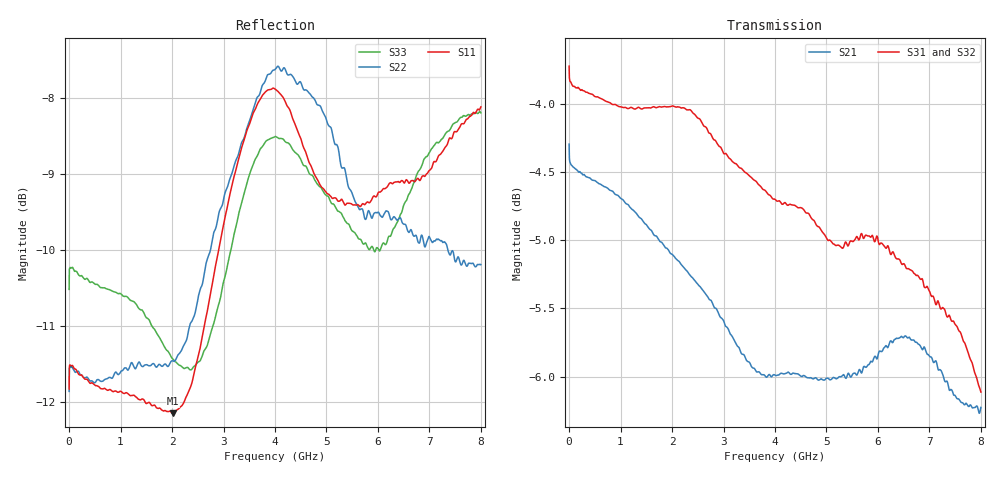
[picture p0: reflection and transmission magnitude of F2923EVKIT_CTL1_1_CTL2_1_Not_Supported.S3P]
! Integrated Device Technology
! Corporate Headquarters
! 6024 Silver Creek Valley Road
! San Jose, CA 95138  USA
! Phone:  1-408-284-8200
! Toll Free:  1-800-223-1366
! Webpage:  http://www.idt.com/
! Timing and RF Division
! 515 Groton Road, Suite 102
! Westford, MA 01886-6024
! Device:  F2923
! Description: Constant Impedance Kz SP2T RF Switch
! Frequency:  0.3 MHz to 8 GHz
! Package:  4 mm x 4 mm QFN Plastic Package: 20 pin
! Ports:  3 RF, 3 DC
!  Pin  1  = GND
!  Pin  2  = GND
!  Pin  3  = RF1  = Port 1
!  Pin  4  = GND
!  Pin  5  = GND
!  Pin  6  = GND
!  Pin  7  = GND
!  Pin  8  = RF_COM  = Port 3
!  Pin  9  = GND
!  Pin  10  = GND
!  Pin  11  = GND
!  Pin  12  = GND
!  Pin  13  = RF2  = Port 2
!  Pin  14  = GND
!  Pin  15  = NC
!  Pin  16  = CTL2
!  Pin  17  = CTL1
!  Pin  18  = NC
!  Pin  19  = ModeCTL
!  Pin  20  = VCC
!  EP  = GND
! State:  Not Supported
! Voltage:  VCC  = +3.3 V
!  CTL1  = 3.3 V (Logic HIGH)
!  CTL2  = 3.3 V (Logic HIGH)
! Data:  The device was measured on the F2923 EVKit
!  using a calibrated network analyzer.
!  The results below include the EVKit RF connector and
!		PCB loss effects. The reference plane is at
!  the SMA coaxial interface. Refer to the separate
!  measured thru line.s2p file for connector and PCB loss
!  and effects.
! Misc:
! Date Measured:  2017-8-14
! Date:  2017-8-14  SPJ
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# Hz S dB R 50
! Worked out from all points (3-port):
!   1601 points, 300 kHz to 8 GHz, reference 50 ohm
!   strongest paths, dB at 300 kHz, 2 GHz, 4 GHz, 6 GHz, 8 GHz:
!     S31: -3.7, -4.0, -4.7, -5.0, -6.1
!     S32: -3.7, -4.2, -4.7, -4.8, -5.5
!     S21: -4.3, -5.1, -6.0, -5.8, -6.2
!   lowest |S11| = -12.2 dB at 2.01 GHz (marker M1), VSWR 1.66, Z = 67.3 - j23.9 ohm
!   |S11| at or under -10 dB: start of sweep to 2.906 GHz
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300000  -11.83 -179.2  -4.30 -0.0  -3.72 0.0
        -4.30 0.0  -11.87 -178.7  -3.73 0.1
        -3.72 -0.0  -3.73 -0.0  -10.52 -179.1
9.252653e8  -11.87 91.5  -4.69 -102.6  -4.00 -98.5
            -4.67 -102.6  -11.62 88.3  -4.06 -99.2
            -4.01 -98.4  -4.06 -99.2  -10.57 96.7
2.010225e9  -12.16 -42.5  -5.06 138.4  -4.02 146.7
            -5.11 138.3  -11.46 -46.1  -4.20 145.5
            -4.01 146.6  -4.18 145.4  -11.44 -28.2
2.570204e9  -11.21 -126.5  -5.41 77.7  -4.12 86.4
            -5.35 77.3  -10.49 -127.7  -4.25 85.4
            -4.13 86.6  -4.25 85.7  -11.43 -110.2
3.175181e9  -9.12 153.2  -5.75 12.4  -4.38 21.9
            -5.71 13.0  -8.97 151.9  -4.44 20.9
            -4.42 21.6  -4.45 20.9  -9.90 163.2
4.00015e9  -7.88 64.3  -5.98 -74.1  -4.70 -64.9
           -5.99 -74.3  -7.62 58.5  -4.73 -66.2
           -4.70 -64.6  -4.74 -66.2  -8.51 71.7
5.010112e9  -9.26 -16.4  -6.05 177.0  -4.95 -171.5
            -6.01 177.0  -8.31 -33.3  -4.91 -172.5
            -4.99 -171.5  -4.91 -172.4  -9.29 -14.2
5.890079e9  -9.32 -85.5  -5.80 82.0  -5.03 94.8
            -5.89 81.7  -9.58 -105.0  -4.78 93.4
            -4.96 95.5  -4.81 93.0  -9.96 -74.9
6.810045e9  -9.09 -166.9  -5.80 -22.2  -5.28 -5.1
            -5.77 -21.8  -9.91 -177.9  -5.02 -7.9
            -5.28 -5.6  -5.01 -8.1  -8.95 -149.1
8e9  -8.12 63.9  -6.27 -158.9  -6.01 -135.9
     -6.23 -159.9  -10.20 54.6  -5.45 -139.7
     -6.11 -134.8  -5.46 -140.2  -8.19 90.2
